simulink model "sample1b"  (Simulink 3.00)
settings: Solver=ode1  SolverMode=SingleTasking  StartTime=0.0  StopTime=70  FixedStep=0.15  MaxStep=0.5  RelTol=1e-1  AbsTol=1e-1

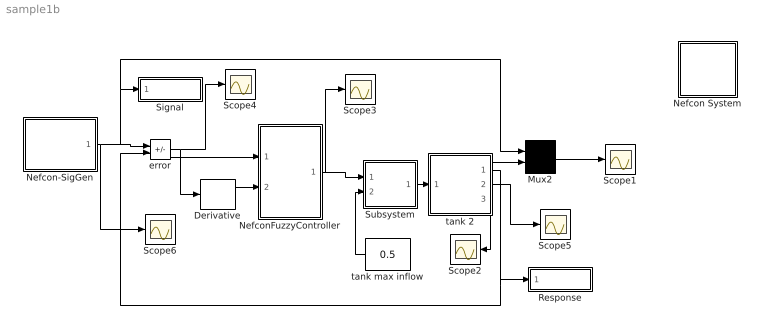
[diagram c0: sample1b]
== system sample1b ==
  Derivative : Derivative
  Mux2 : Mux  Inputs=2
  Nefcon System : Subsystem
  Nefcon-SigGen : Subsystem
  NefconFuzzyController : Subsystem
  Response : Subsystem
  Scope{1..6} (6 alike) : Scope
  Signal : Subsystem
  Subsystem : Subsystem  mask(Valve){}
      mask help: Valve
      mask init:
      | InitialPosition = @1;
  error : Sum  Inputs=+-  SaturateOnIntegerOverflow=on
  tank 2 : Subsystem  mask(Water tank){}
      mask help: Cylindrical water tank with overflow signal
      mask init:
      | ht=@1;area=@2;outletArea=@3;overflowLimit=@4;initialHt=@5;
  tank max inflow : Constant  Orientation=left  Value=0.5
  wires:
  Mux2/1 -> Scope1/1
  error/1 -> Derivative/1, Scope4/1, NefconFuzzyController/1(in_1)
  NefconFuzzyController/1(out_1) -> Scope3/1, Subsystem/1(control)
  tank 2/1(water level) -> Response/1(In1), error/2, Mux2/2
  Derivative/1 -> NefconFuzzyController/2(in_2)
  tank max inflow/1 -> Subsystem/2(source flow)
  Subsystem/1(out flow) -> tank 2/1(flow in)
  tank 2/3(overflow flag) -> Scope2/1
  tank 2/2(flow out) -> Scope5/1
  Nefcon-SigGen/1(out_1) -> Signal/1(In1), Mux2/1, error/1, Scope6/1

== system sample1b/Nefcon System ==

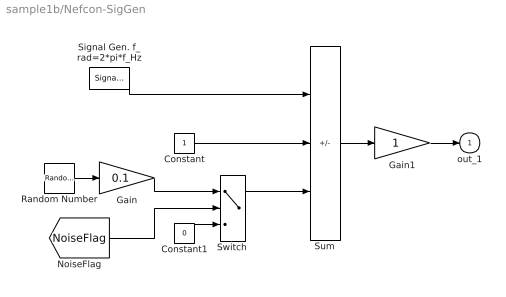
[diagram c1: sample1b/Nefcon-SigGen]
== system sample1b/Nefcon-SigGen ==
  Constant : Constant  Value=1
  Constant1 : Constant  Value=0
  Gain : Gain  Gain=0.1  SaturateOnIntegerOverflow=on
  Gain1 : Gain  Gain=1  SaturateOnIntegerOverflow=on
  Random Number : RandomNumber  Mean=0  Variance=1  Seed=0  SampleTime=0
  Signal Gen. f_rad=2*pi*f_Hz : SignalGenerator  WaveForm=square  Amplitude=0.500000  Frequency=0.100000  Units=rad/sec
  Sum : Sum  Inputs=-++  SaturateOnIntegerOverflow=on
  Switch : Switch  Threshold=0.5
  out_1 : Outport  Port=1
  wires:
  Constant1/1 -> Switch/3
  Sum/1 -> Gain1/1
  Gain1/1 -> out_1/1
  Signal Gen. f_rad=2*pi*f_Hz/1 -> Sum/1
  Constant/1 -> Sum/2
  Gain/1 -> Switch/1
  Random Number/1 -> Gain/1
  Switch/1 -> Sum/3
  [NoiseFlag] -> Switch/2

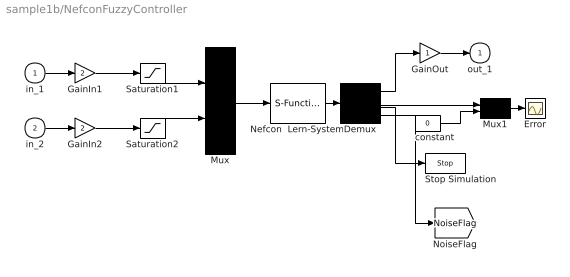
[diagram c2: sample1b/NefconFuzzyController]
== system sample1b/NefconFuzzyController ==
  in_1 : Inport  Port=1  PortWidth=-1  SampleTime=-1  DataType=auto
  in_2 : Inport  Port=2  PortWidth=-1  SampleTime=-1  DataType=auto
  Demux : Demux  Outputs=4
  Error : Scope
  GainIn1 : Gain  Gain=2  SaturateOnIntegerOverflow=on
  GainIn2 : Gain  Gain=2  SaturateOnIntegerOverflow=on
  GainOut : Gain  Gain=1  SaturateOnIntegerOverflow=on
  Mux : Mux  Inputs=2
  Mux1 : Mux  Inputs=2
  Nefcon  Lern-System : S-Function  FunctionName=snefcon  PortCounts=[]  SFunctionModules=''
  Saturation1 : Saturate  UpperLimit=1  LowerLimit=-1
  Saturation2 : Saturate  UpperLimit=1  LowerLimit=-1
  Stop Simulation : Stop
  constant : Constant  Value=0
  out_1 : Outport  Port=1
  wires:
  Demux/4 -> [NoiseFlag]
  constant/1 -> Mux1/2
  Demux/3 -> Stop Simulation/1
  Mux1/1 -> Error/1
  Demux/2 -> Mux1/1
  GainOut/1 -> out_1/1
  Demux/1 -> GainOut/1
  Nefcon  Lern-System/1 -> Demux/1
  Mux/1 -> Nefcon  Lern-System/1
  Saturation2/1 -> Mux/2
  GainIn2/1 -> Saturation2/1
  in_2/1 -> GainIn2/1
  Saturation1/1 -> Mux/1
  GainIn1/1 -> Saturation1/1
  in_1/1 -> GainIn1/1

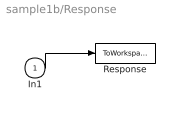
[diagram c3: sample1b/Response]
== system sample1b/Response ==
  In1 : Inport  Port=1  PortWidth=-1  SampleTime=-1  DataType=auto
  Response : ToWorkspace  VariableName=nef_y  SampleTime=0  SaveFormat=Matrix
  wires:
  In1/1 -> Response/1

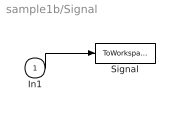
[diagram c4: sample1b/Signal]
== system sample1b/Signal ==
  In1 : Inport  Port=1  PortWidth=-1  SampleTime=-1  DataType=auto
  Signal : ToWorkspace  VariableName=nef_u  SampleTime=0  SaveFormat=Matrix
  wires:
  In1/1 -> Signal/1

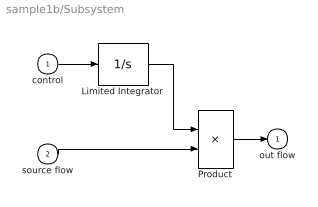
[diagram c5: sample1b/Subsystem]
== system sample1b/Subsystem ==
  control : Inport  Port=1  PortWidth=-1  SampleTime=-1  DataType=auto
  source flow : Inport  Port=2  PortWidth=-1  SampleTime=-1  DataType=auto
  Limited Integrator : Integrator  ExternalReset=none  InitialConditionSource=internal  InitialCondition=InitialPosition  LimitOutput=on  UpperSaturationLimit=1  LowerSaturationLimit=0  ShowSaturationPort=off  ShowStatePort=off  AbsoluteTolerance=auto
  Product : Product  Inputs=2  SaturateOnIntegerOverflow=on
  out flow : Outport  Port=1
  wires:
  source flow/1 -> Product/2
  Product/1 -> out flow/1
  control/1 -> Limited Integrator/1
  Limited Integrator/1 -> Product/1

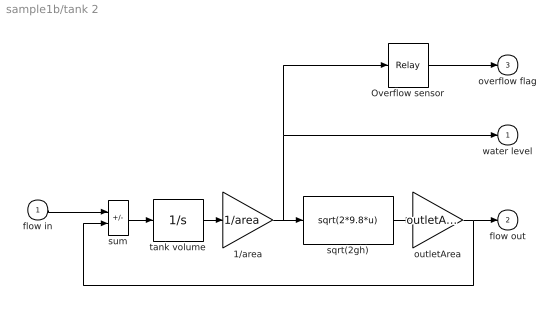
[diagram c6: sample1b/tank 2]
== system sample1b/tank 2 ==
  flow in : Inport  Port=1  PortWidth=-1  SampleTime=-1  DataType=auto
  1/area : Gain  Gain=1/area  SaturateOnIntegerOverflow=on
  Overflow sensor : Relay  OnSwitchValue=ht - overflowLimit  OffSwitchValue=ht - overflowLimit  OnOutputValue=1  OffOutputValue=0
  outletArea : Gain  Gain=outletArea  SaturateOnIntegerOverflow=on
  sqrt(2gh) : Fcn  Expr=sqrt(2*9.8*u)
  sum : Sum  Inputs=+-  SaturateOnIntegerOverflow=on
  tank volume : Integrator  ExternalReset=none  InitialConditionSource=internal  InitialCondition=initialHt * area  LimitOutput=on  UpperSaturationLimit=ht * area  LowerSaturationLimit=0  ShowSaturationPort=off  ShowStatePort=off  AbsoluteTolerance=auto
  water level : Outport  Port=1
  flow out : Outport  Port=2
  overflow flag : Outport  Port=3
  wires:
  1/area/1 -> water level/1, Overflow sensor/1, sqrt(2gh)/1
  outletArea/1 -> sum/2, flow out/1
  sqrt(2gh)/1 -> outletArea/1
  tank volume/1 -> 1/area/1
  Overflow sensor/1 -> overflow flag/1
  flow in/1 -> sum/1
  sum/1 -> tank volume/1
